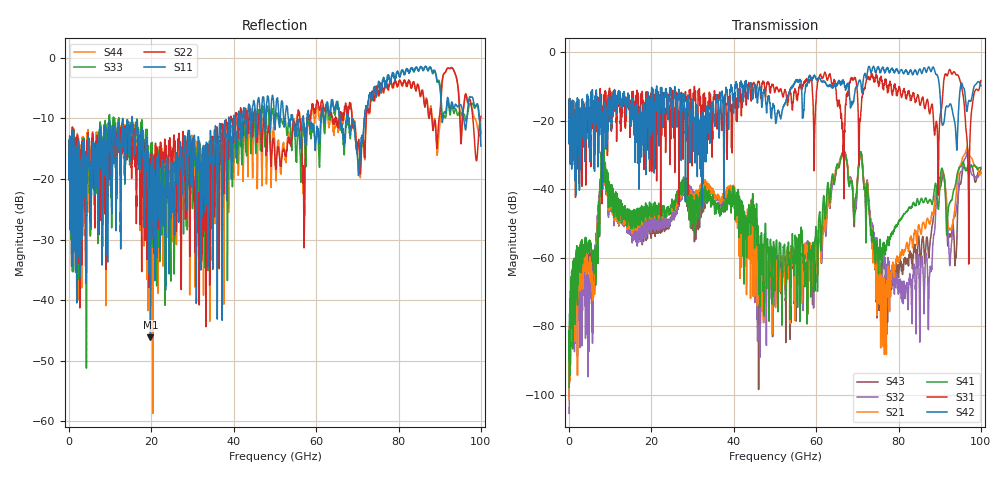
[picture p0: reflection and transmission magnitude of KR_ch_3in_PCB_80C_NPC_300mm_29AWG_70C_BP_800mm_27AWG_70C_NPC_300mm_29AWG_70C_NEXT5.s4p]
# GHz S RI R 45
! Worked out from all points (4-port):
!   4000 points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, 25 MHz to 100 GHz, reference 45 ohm
!   strongest paths, dB at 25 MHz, 25.02 GHz, 50.02 GHz, 75.03 GHz, 100 GHz:
!     S42: -20.0, -17.9, -18.0, -4.4, -9.7
!     S31: -20.0, -12.2, -11.3, -8.6, -8.3
!     S41: -97.7, -43.5, -66.2, -58.2, -33.6
!     S21: -101.4, -45.0, -62.8, -64.7, -35.0
!     S32: -105.3, -47.1, -74.1, -57.2, -35.3
!     S43: -100.1, -46.7, -69.8, -64.7, -34.1
!   lowest |S11| = -46.1 dB at 19.77 GHz (marker M1), VSWR 1.01, Z = 45.4 + j0.0365 ohm
!   |S11| at or under -10 dB: start of sweep to 15.33 GHz; 15.36 GHz to 38.77 GHz (23.42 GHz wide, 86.5 % of centre); 67.96 GHz to 71.67 GHz (3.712 GHz wide, 5.32 % of centre)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
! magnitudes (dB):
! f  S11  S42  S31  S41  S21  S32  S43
! 25 MHz  -16.0  -20.0  -20.0  -97.7  -101.4  -105.3  -100.1
! 8.275 GHz  -15.0  -18.2  -16.8  -30.5  -31.0  -31.3  -30.9
! 19.77 GHz  -46.1  -15.3  -15.0  -46.6  -48.0  -50.8  -50.5
! 55.08 GHz  -13.0  -8.0  -11.3  -58.1  -61.9  -60.0  -69.6
! 70.8 GHz  -15.4  -8.8  -18.6  -29.0  -29.9  -29.6  -29.1
! 76.75 GHz  -4.8  -5.6  -7.8  -57.6  -67.9  -60.4  -65.1
! 100 GHz  -14.6  -9.7  -8.3  -33.6  -35.0  -35.3  -34.1
